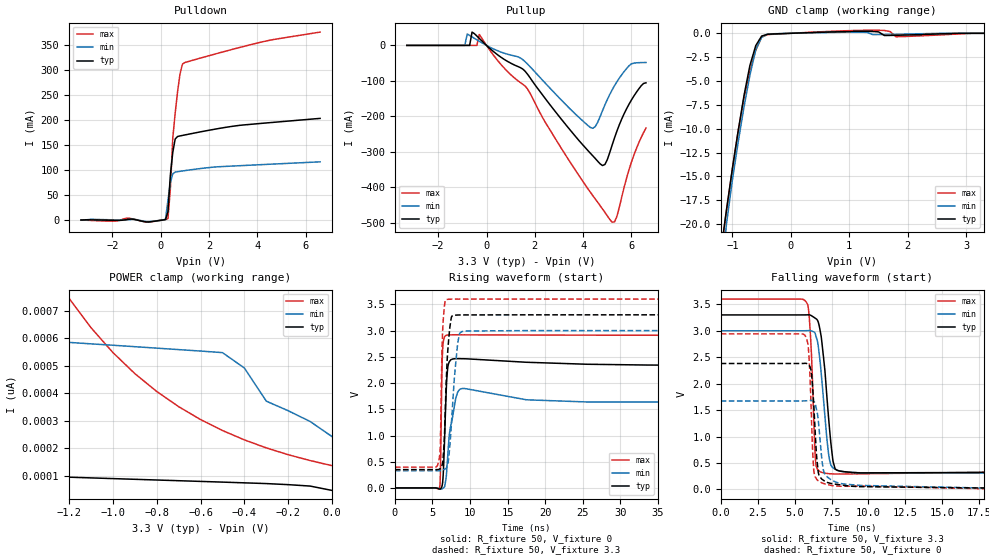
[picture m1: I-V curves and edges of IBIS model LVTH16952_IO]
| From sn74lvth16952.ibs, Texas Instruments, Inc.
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|   Model LVTH16952  I/O
[Model]   LVTH16952_IO
|Signals
Model_type  I/O
Polarity   Non-Inverting
Enable   Active-Low
Vinl = 0.8V
Vinh = 2.0V
Vmeas= 1.5V
Cref = 50pf
Rref = 500
Vref = 0V
| variable   typ   min   max
C_comp   10p   NA   NA
[Temperature Range]   50   100   0
[Voltage range]   3.3   3   3.6
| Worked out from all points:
|   slope of the pulldown table from 0 to 0.495 V, typ, clamps not added: 3.71 ohm
|   slope of the pullup table from 0 to 0.495 V, typ, clamps not added: 17.5 ohm
|   GND clamp passes 1 mA (typ) near -0.57 V on its own axis
|   rising waveform, R_fixture 50, V_fixture 0: 20-80 % time 336ps typ, 733ps min, 180ps max; typ from 0.006 V to 2.33 V
|   falling waveform, R_fixture 50, V_fixture 3.3: 20-80 % time 560ps typ, 516ps min, 271ps max; typ from 3.3 V to 0.339 V
|   rising waveform, R_fixture 50, V_fixture 3.3: 20-80 % time 510ps typ, 807ps min, 266ps max; typ from 0.354 V to 3.3 V
|   falling waveform, R_fixture 50, V_fixture 0: 20-80 % time 314ps typ, 389ps min, 239ps max; typ from 2.38 V to 0.007 V
|Process range|   weak   strong
[Pullup]
|   50C:3.3V:   100C:3V:weak   0C:3.6V:strong
|   Voltage   I(typ)   I(min)   I(max)
-3.3V     75.07uA    45.68uA    127uA
-700mV    61.35uA    28.17mA    114.9uA
-600mV    37.62mA    24.03mA    113.5uA
-400mV    26.47mA    15.78mA    74.09uA
-300mV    19.78mA    11.73mA    30.86mA
1.5V      -66.61mA   -40.04mA   -109.4mA
4.3V      -304.2mA   -231.5mA   -414.2mA
4.8V      -338.8mA   -184.2mA   -461.2mA
5.2V      -281.1mA   -125.4mA   -498.6mA
5.4V      -241.2mA   -102.2mA   -481.6mA
5.9V      -165.6mA   -57.31mA   -350.2mA
6.6V      -105.4mA   -48.12mA   -233.1mA
[Pulldown]
|   50C:3.3V:   100C:3V:weak   0C:3.6V:strong
|   Voltage   I(typ)   I(min)   I(max)
-3.3V     367.5uA    615.7uA    301.1uA
-500mV    -3.467mA   -2.8mA     -3.941mA
100mV     551.2uA    517.4uA    569.2uA
200mV     1.371mA    2.105mA    1.37mA
300mV     17mA       39.92mA    3.286mA
400mV     90.44mA    74.64mA    62.84mA
500mV     135.6mA    92.86mA    164.2mA
600mV     162.5mA    96.18mA    214.3mA
800mV     168.6mA    97.78mA    292.5mA
900mV     169.6mA    98.49mA    312.1mA
4.1V      193.4mA    111mA      355.5mA
6.6V      203.7mA    116.7mA    376.2mA
[GND Clamp]
|   50C:3.3V:   100C:3V:weak   0C:3.6V:strong
|   Voltage   I(typ)   I(min)   I(max)
-3.3V     -727.1mA   -676.9mA   -803.5mA
-1.2V     -22.99mA   -26.09mA   -23.15mA
-1.1V     -18.45mA   -19.94mA   -18.59mA
-900mV    -10.2mA    -11.38mA   -10.2mA
-800mV    -6.484mA   -7.675mA   -6.702mA
-700mV    -3.358mA   -4.379mA   -3.927mA
-600mV    -1.288mA   -1.721mA   -1.774mA
-500mV    -289.7uA   -424.4uA   -406.1uA
1.2V      199.7uA    118.8uA    309.4uA
1.6V      -230.1uA   -124.8uA   297.4uA
1.8V      -209uA     -104uA     -357.9uA
3.3V      47.05pA    371.5pA    -3.18nA
[POWER Clamp]
|   50C:3.3V:   100C:3V:weak   0C:3.6V:strong
|   Voltage   I(typ)   I(min)   I(max)
-3.3V     152.2pA    695.8pA    23.56nA
-1.2V     95.25pA    585.1pA    745.3pA
-1.1V     92.68pA    579.7pA    638.7pA
-1V       90.11pA    574.7pA    548.3pA
-900mV    87.55pA    569.5pA    471.7pA
-800mV    84.99pA    564.2pA    406.8pA
-700mV    82.46pA    558.9pA    351.6pA
-500mV    77.34pA    547.9pA    264.8pA
-400mV    74.69pA    491.9pA    230.8pA
-300mV    72.02pA    371.5pA    201.7pA
-100mV    62.94pA    297.6pA    155.7pA
0V        47.05pA    242.6pA    137.1pA
[ramp]
| variable   typ   min   max
dV/dt_r   1.4902E+00/3.6046E-10  1.1506E+00/9.4895E-10  1.7612E+00/1.7919E-10
dV/dt_f   1.7938E+00/5.6470E-10  1.6148E+00/5.2030E-10  1.9846E+00/2.7493E-10
[Rising Waveform]
R_fixture = 50
V_fixture = 0
V_fixture_min = 0
V_fixture_max = 0
L_fixture = 0nH
C_fixture = 0pF
|   50C:3.3V:   100C:3V:weak   0C:3.6V:strong
|   Time   V(typ)   V(min)   V(max)
0s        5.563mV    4.129mV    7.568mV
5.95ns    -16.29mV   -13.02mV   18.44mV
6.05ns    -13.9mV    -17.93mV   232.5mV
6.3ns     56.51mV    -8.883mV   2.459V
6.5ns     460.6mV    10.53mV    2.832V
6.8ns     1.719V     175.6mV    2.908V
7.2ns     2.392V     957.9mV    2.918V
8.1ns     2.466V     1.711V     2.919V
8.95ns    2.465V     1.897V     2.919V
50ns      2.334V     1.641V     2.91V
[Falling Waveform]
R_fixture = 50
V_fixture = 3.3
V_fixture_min = 3
V_fixture_max = 3.6
L_fixture = 0nH
C_fixture = 0pF
|   50C:3.3V:   100C:3V:weak   0C:3.6V:strong
|   Time   V(typ)   V(min)   V(max)
0s        3.3V       3V         3.6V
5.8ns     3.301V     3.002V     3.539V
5.95ns    3.302V     3.004V     3.387V
6.1ns     3.292V     3.002V     2.785V
6.45ns    3.227V     2.897V     453.2mV
6.9ns     2.646V     1.889V     318.6mV
7.3ns     1.356V     671.7mV    298.9mV
7.6ns     535.3mV    409.9mV    295mV
8.05ns    348.6mV    350mV      293.6mV
50ns      338.8mV    329.5mV    390.4mV
[Rising Waveform]
R_fixture = 50
V_fixture = 3.3
V_fixture_min = 3
V_fixture_max = 3.6
L_fixture = 0nH
C_fixture = 0pF
|   50C:3.3V:   100C:3V:weak   0C:3.6V:strong
|   Time   V(typ)   V(min)   V(max)
0s        354.3mV    334mV      400.9mV
5.7ns     354.4mV    333.1mV    441.6mV
6.05ns    377.7mV    336.5mV    847.4mV
6.25ns    423.9mV    342.9mV    2.514V
6.4ns     533.8mV    348.3mV    3.118V
6.85ns    2.091V     380.4mV    3.591V
7.5ns     3.241V     1.177V     3.598V
8.35ns    3.296V     2.745V     3.599V
8.85ns    3.298V     2.977V     3.599V
50ns      3.3V       3V         3.6V
[Falling Waveform]
R_fixture = 50
V_fixture = 0
V_fixture_min = 0
V_fixture_max = 0
L_fixture = 0nH
C_fixture = 0pF
|   50C:3.3V:   100C:3V:weak   0C:3.6V:strong
|   Time   V(typ)   V(min)   V(max)
0s        2.382V     1.674V     2.942V
5.7ns     2.385V     1.675V     2.916V
5.95ns    2.353V     1.682V     2.614V
6.15ns    2.176V     1.682V     1.277V
6.3ns     1.588V     1.66V      350.1mV
6.45ns    795.8mV    1.554V     214.8mV
6.6ns     323.3mV    1.319V     165.7mV
6.95ns    174.7mV    368.3mV    112.9mV
7.55ns    110.6mV    172.1mV    73.46mV
50ns      6.83mV     6.179mV    8.497mV
